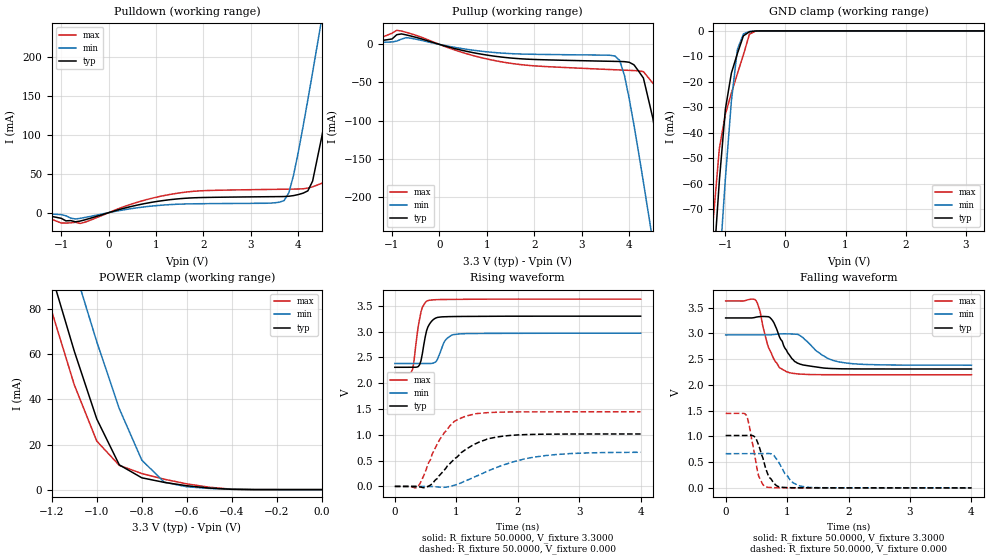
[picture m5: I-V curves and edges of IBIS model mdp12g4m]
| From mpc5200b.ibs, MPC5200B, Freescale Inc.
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|   Model mdp12g4m
[Model]   mdp12g4m
Model_type   I/O
Polarity   Non-Inverting
Enable   Active-High
Vinl =   0.8000V
Vinh =   2.0000V
Vmeas =   1.5000V
C_comp   2.1096pF   1.4802pF   2.7108pF
[Temperature Range]   27.0000   0.1250k   -40.0000
[Voltage Range]   3.3000V   2.9700V   3.6300V
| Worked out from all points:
|   slope of the pulldown table from 0 to 0.495 V, typ, clamps not added: 60 ohm
|   slope of the pullup table from 0 to 0.495 V, typ, clamps not added: 61.6 ohm
|   GND clamp passes 1 mA (typ) near -0.64 V on its own axis
|   POWER clamp passes 1 mA (typ) near -0.53 V on its own axis
|   rising waveform, R_fixture 50.0000, V_fixture 3.3000: 20-80 % time 106ps typ, 130ps min, 103ps max; typ from 2.31 V to 3.3 V
|   rising waveform, R_fixture 50.0000, V_fixture 0.000: 20-80 % time 570ps typ, 892ps min, 387ps max; typ from 0 V to 1.02 V
|   falling waveform, R_fixture 50.0000, V_fixture 3.3000: 20-80 % time 257ps typ, 376ps min, 219ps max; typ from 3.3 V to 2.31 V
|   falling waveform, R_fixture 50.0000, V_fixture 0.000: 20-80 % time 171ps typ, 214ps min, 133ps max; typ from 1.02 V to 0 V
[Pulldown]
| voltage   I(typ)   I(min)   I(max)
-3.3V     -520.3uA   -427.6uA   -409.9uA
-600mV    -10.77mA   -7.285mA   -13.83mA
1.3V      16.74mA    10.4mA     23.5mA
3.7V      20.76mA    15.59mA    30.15mA
3.9V      21.99mA    48.6mA     30.33mA
4.2V      28.07mA    145.2mA    31.61mA
4.3V      40.53mA    180.2mA    33.2mA
4.5V      99.48mA    251.9mA    37.97mA
4.7V      169.7mA    324.8mA    52.04mA
4.9V      242.9mA    398.5mA    109.3mA
5.3V      393.7mA    547.3mA    257.2mA
6.6V      899.4mA    1.04A      765.5mA
[Pullup]
| voltage   I(typ)   I(min)   I(max)
-3.3V     1.028mA    1.577mA    988uA
-1.5V     2.453mA    2.019mA    2.101mA
-900mV    12.73mA    4.365mA    18.52mA
1.3V      -16.57mA   -11.35mA   -22.82mA
3.7V      -22.3mA    -15.28mA   -33.3mA
3.9V      -22.65mA   -40.84mA   -33.84mA
4.3V      -44.28mA   -181mA     -35.83mA
4.5V      -97.27mA   -259.4mA   -51.01mA
4.7V      -171.5mA   -339.3mA   -67.06mA
4.9V      -250.2mA   -420.1mA   -104.9mA
5.3V      -411.9mA   -583.3mA   -256.4mA
6.6V      -948.9mA   -1.12A     -792.6mA
[GND_clamp]
| voltage   I(typ)   I(min)   I(max)
-3.3V     -948.1mA   -982.8mA   -929.6mA
-1.3V     -130.7mA   -168mA     -108.8mA
-1.2V     -93.35mA   -129.8mA   -73.5mA
-1.1V     -58.65mA   -92.83mA   -45.99mA
-1V       -30.69mA   -57.94mA   -32.68mA
-900mV    -16.54mA   -27.44mA   -24.36mA
-800mV    -8.854mA   -7.262mA   -16.75mA
-700mV    -1.936mA   -1.183mA   -9.358mA
-600mV    -366uA     -212.8uA   -1.293mA
-500mV    -39.22uA   -34.56uA   -92.73uA
3.3V      541.3pA    33.88uA    287.7pA
[POWER_clamp]
| voltage   I(typ)   I(min)   I(max)
-3.3V     897.6mA    912.2mA    893.7mA
-1.3V     130.2mA    167.4mA    114.6mA
-1.2V     95.06mA    132.3mA    79.13mA
-1.1V     61.46mA    98.2mA     46.53mA
-1V       31.32mA    65.57mA    21.52mA
-900mV    10.96mA    35.88mA    10.75mA
-800mV    5.231mA    13.06mA    7.129mA
-700mV    3.197mA    3.28mA     4.595mA
-600mV    1.712mA    1.263mA    2.547mA
-500mV    672.1uA    514.1uA    1.035mA
-400mV    127.3uA    134.7uA    183.8uA
0V        541.3pA    4.807nA    325.5pA
[Ramp]
| variable   typ   min   max
dV/dt_r   0.6043/0.5535n   0.3320/0.6730n   0.8671/0.3826n
dV/dt_f   0.5944/0.2577n   0.3417/0.3472n   0.8598/0.2216n
R_load = 50.0000
[Rising Waveform]
R_fixture = 50.0000
V_fixture = 3.3000
V_fixture_min = 2.9700
V_fixture_max = 3.6300
| time   V(typ)   V(min)   V(max)
0s        2.309V     2.382V     2.197V
269.4ps   2.309V     2.382V     2.216V
291.8ps   2.31V      2.382V     2.277V
381.6ps   2.323V     2.383V     3.109V
426.5ps   2.44V      2.383V     3.386V
538.8ps   3.092V     2.382V     3.601V
673.5ps   3.267V     2.423V     3.62V
830.6ps   3.29V      2.847V     3.624V
987.8ps   3.293V     2.948V     3.627V
4ns       3.3V       2.97V      3.63V
[Rising Waveform]
R_fixture = 50.0000
V_fixture = 0.000
| time   V(typ)   V(min)   V(max)
0s        94.79nV    267.5nV    252.4nV
359.2ps   -2.313mV   29.43uV    -17.35mV
426.5ps   -14.3mV    275.9uV    93.02mV
561.2ps   11.9mV     365.8uV    483.5mV
808.2ps   321.5mV    -17.03mV   1.047V
965.3ps   523.8mV    20.62mV    1.258V
1.167ns   727.3mV    115.6mV    1.367V
1.504ns   920mV      294.1mV    1.429V
2.204ns   1.008V     556.5mV    1.445V
4ns       1.016V     661.7mV    1.446V
[Falling Waveform]
R_fixture = 50.0000
V_fixture = 3.3000
V_fixture_min = 2.9700
V_fixture_max = 3.6300
| time   V(typ)   V(min)   V(max)
0s        3.3V       2.97V      3.63V
493.9ps   3.315V     2.97V      3.637V
561.2ps   3.327V     2.97V      3.425V
673.5ps   3.326V     2.969V     2.818V
763.3ps   3.25V      2.976V     2.556V
1.033ns   2.589V     2.99V      2.239V
1.257ns   2.387V     2.92V      2.206V
1.571ns   2.33V      2.577V     2.198V
1.886ns   2.312V     2.437V     2.197V
4ns       2.309V     2.382V     2.197V
[Falling Waveform]
R_fixture = 50.0000
V_fixture = 0.000
| time   V(typ)   V(min)   V(max)
0s        1.016V     663.8mV    1.446V
336.7ps   1.016V     663.9mV    1.411V
471.4ps   991.7mV    663.6mV    645.3mV
538.8ps   825mV      663.5mV    224.3mV
651ps     376mV      666mV      22.65mV
763.3ps   126.6mV    653.3mV    4.163mV
853.1ps   26.43mV    519.1mV    1.892mV
1.055ns   3.243mV    137.3mV    465.2uV
1.28ns    1.025mV    19.36mV    97.45uV
4ns       882.7nV    1.02uV     1.495uV
